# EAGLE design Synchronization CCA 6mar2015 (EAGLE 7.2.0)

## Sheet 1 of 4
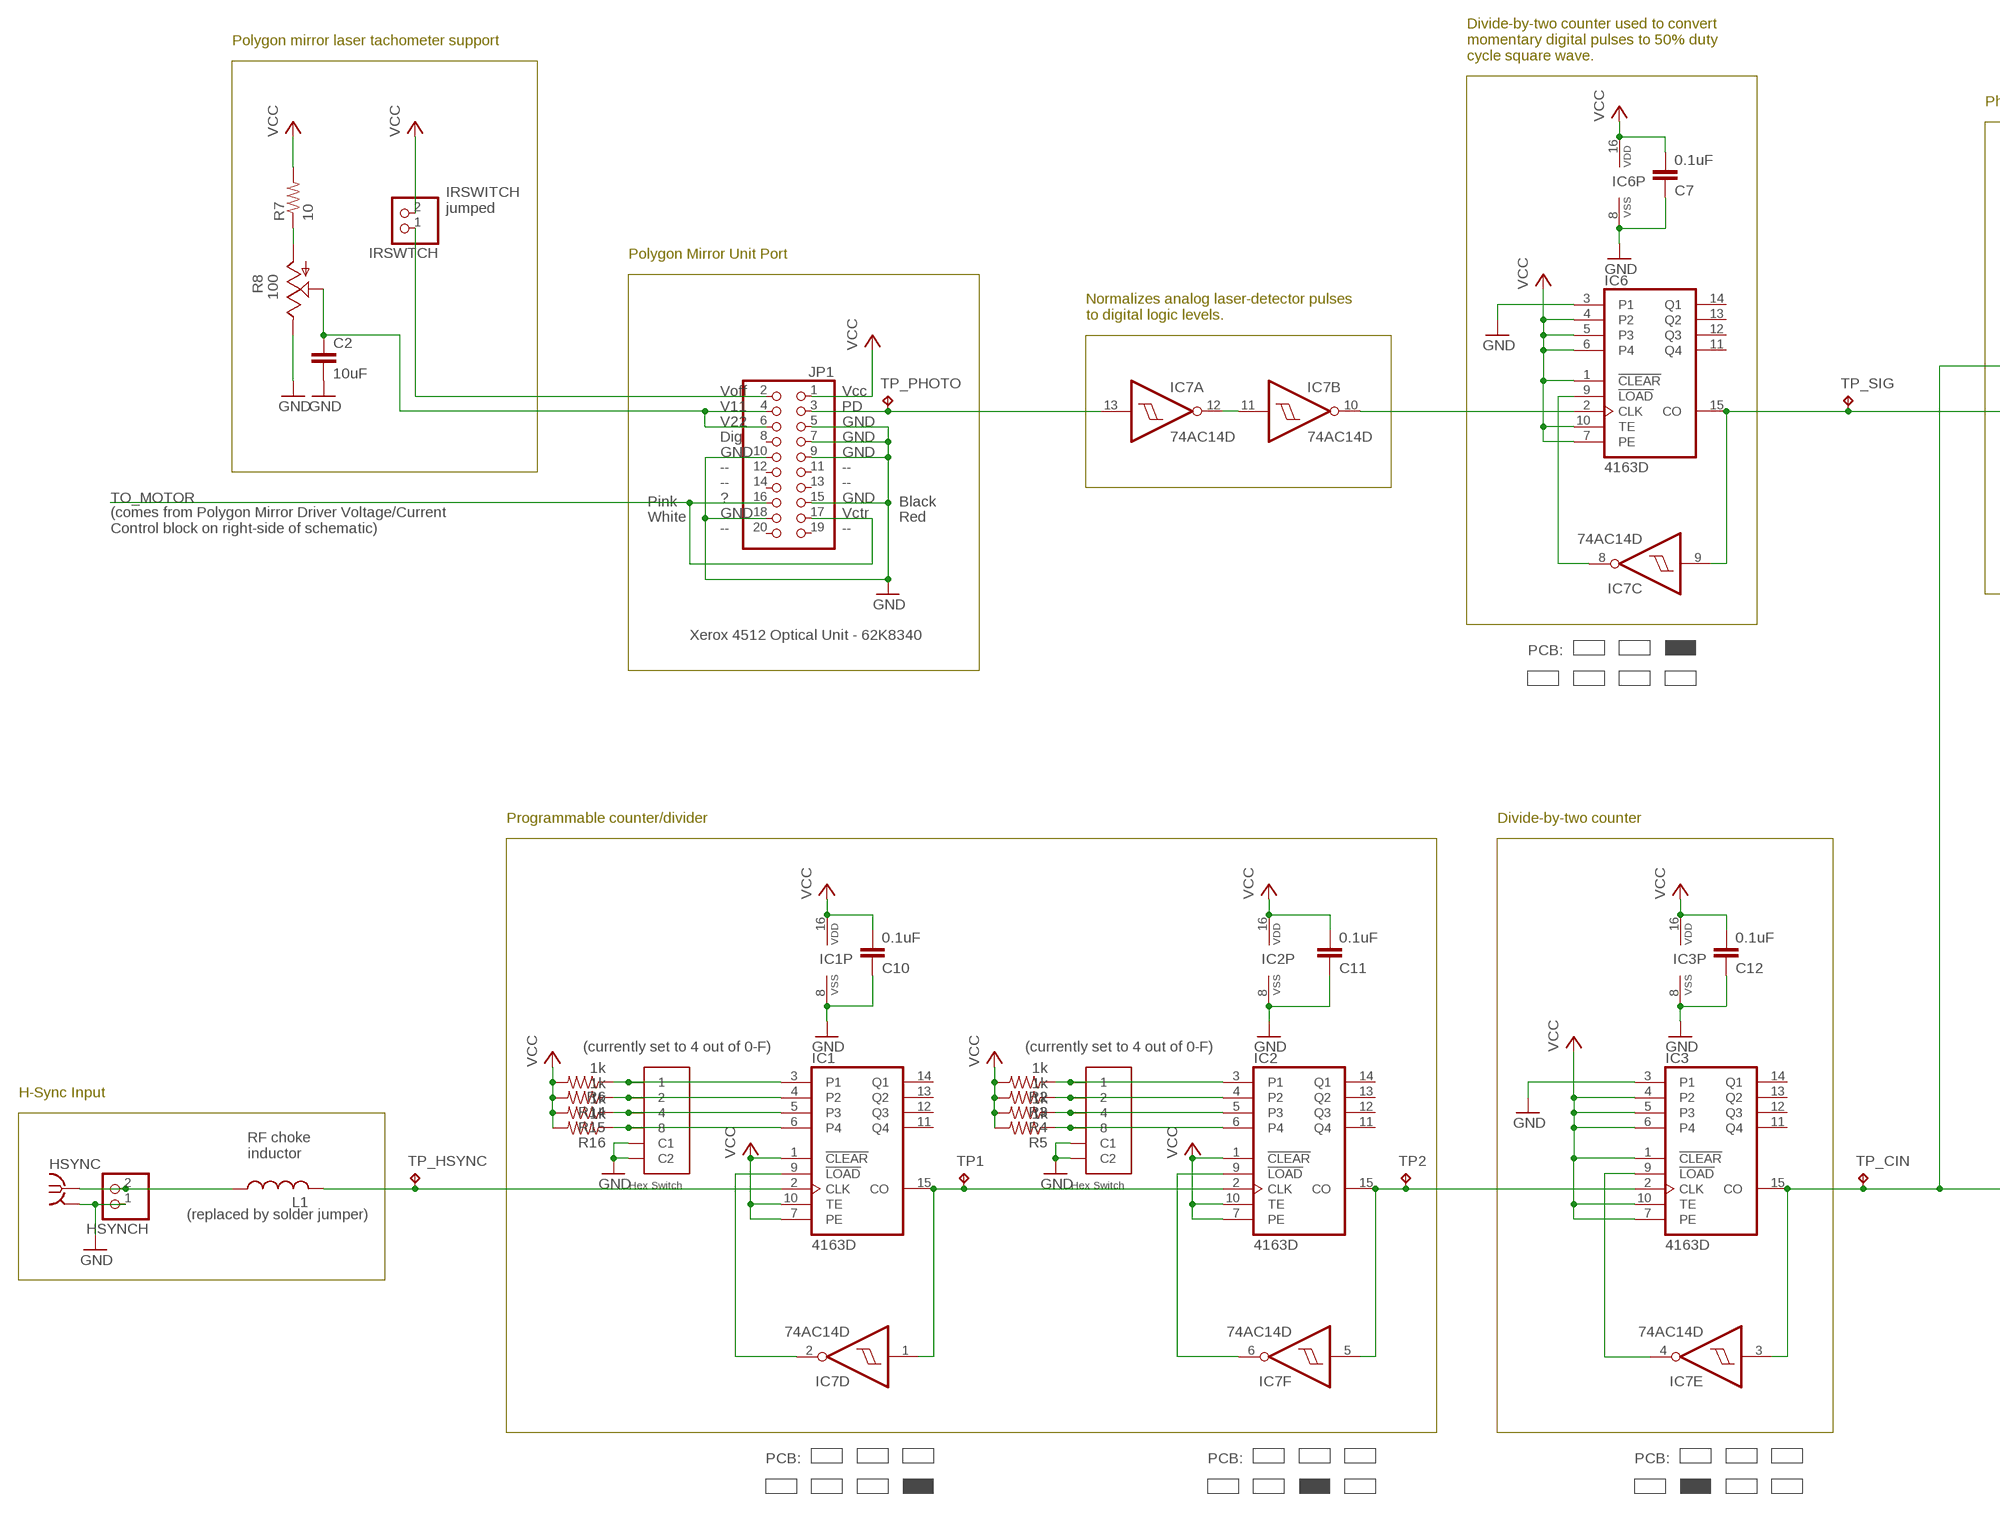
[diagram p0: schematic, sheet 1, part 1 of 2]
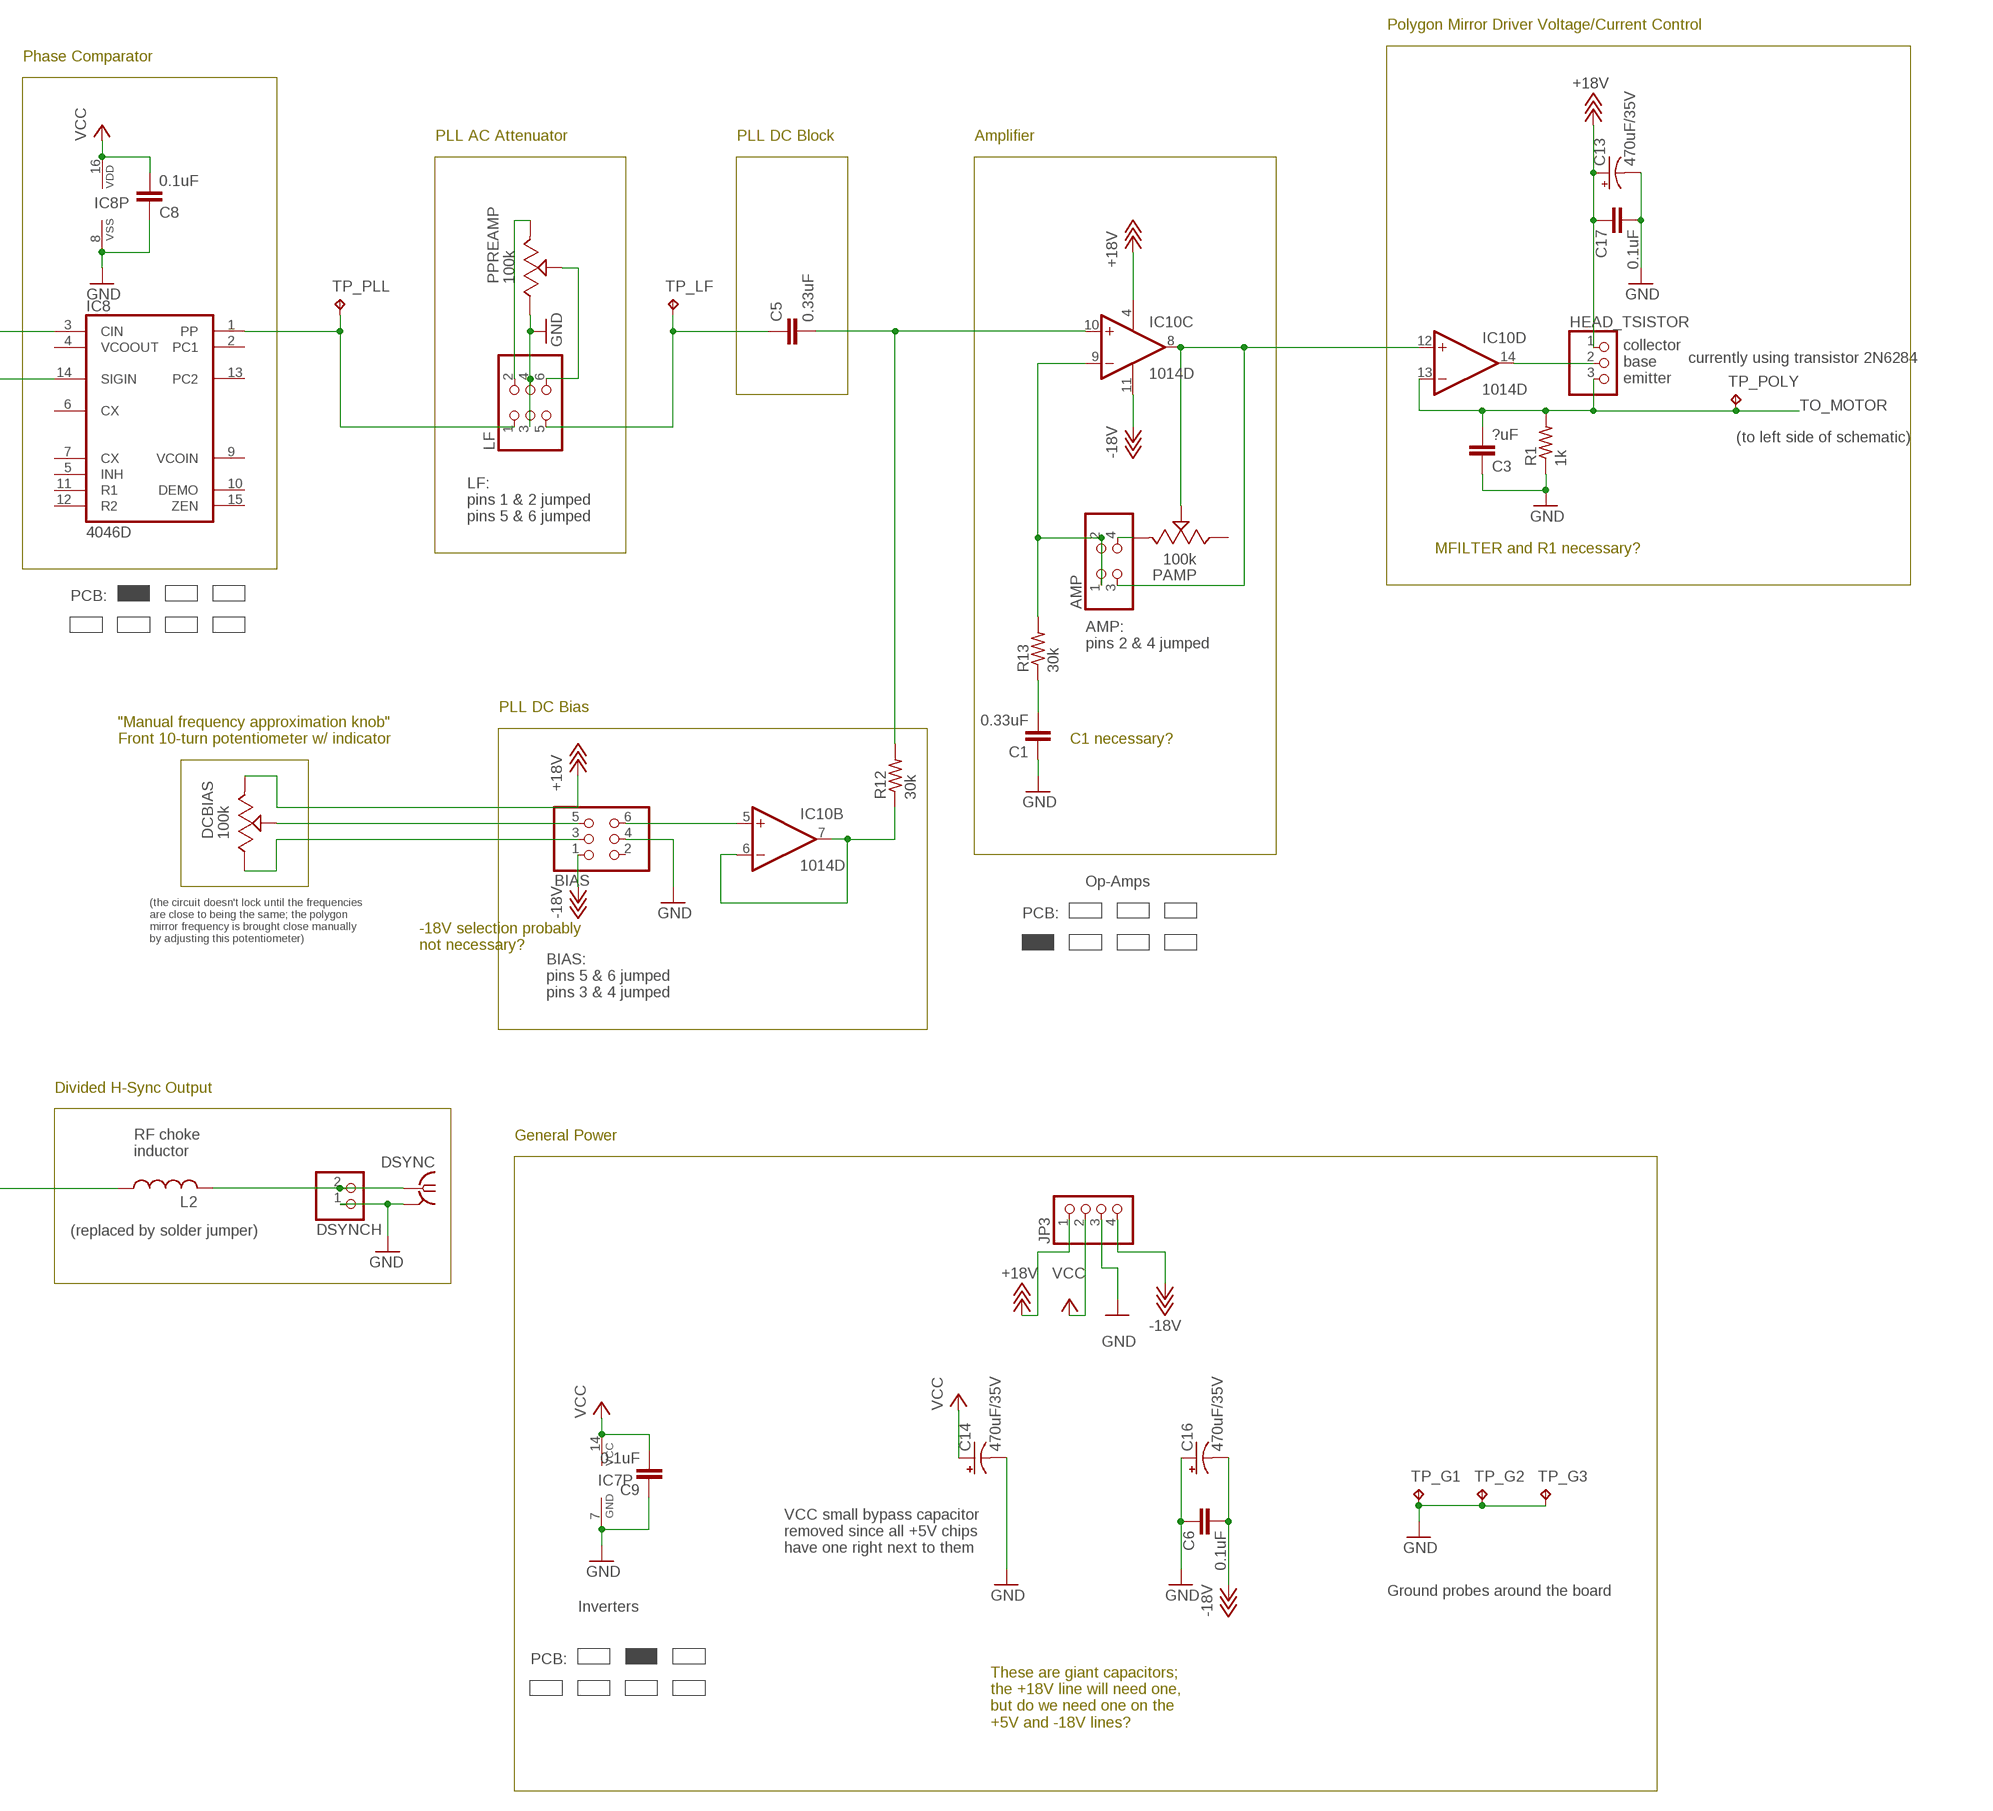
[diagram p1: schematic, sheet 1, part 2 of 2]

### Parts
AMP  PINHD-2X2  [2X02]
BIAS  PINHD-2X3  [2X03]
C1  0.33uF  C-EUC0805  [C0805]
C2  10uF  C-EUC0805  [C0805]
C3  ?uF  C-EUC0805  [C0805]
C5  0.33uF  C-EUC0805  [C0805]
C6  0.1uF  C-EUC0805  [C0805]
C7  0.1uF  C-EUC0805  [C0805]
C8  0.1uF  C-EUC0805  [C0805]
C9  0.1uF  C-EUC0805  [C0805]
C10  0.1uF  C-EUC0805  [C0805]
C11  0.1uF  C-EUC0805  [C0805]
C12  0.1uF  C-EUC0805  [C0805]
C13  470uF/35V  CPOL-USE5-10.5  [E5-10,5]
C14  470uF/35V  CPOL-USE5-10.5  [E5-10,5]
C16  470uF/35V  CPOL-USE5-10.5  [E5-10,5]
C17  0.1uF  C-EUC0805  [C0805]
DCBIAS  100k  POT3352  [POT3352]
DSYNC  SMA-142-0701-801/806  [J502-ND-142-0701-801/806]
DSYNCH  PINHD-1X2  [1X02]
HEAD_TSISTOR  PINHD-1X3  [1X03]
HEX1  HEXROTARY  [HEXROTARYP]
HEX2  HEXROTARY  [HEXROTARYP]
HSYNC  SMA-142-0701-801/806  [J502-ND-142-0701-801/806]
HSYNCH  PINHD-1X2  [1X02]
IC1  4163D  [SO16]
IC2  4163D  [SO16]
IC3  4163D  [SO16]
IC6  4163D  [SO16]
IC7  74AC14D  [SO14]
IC8  4046D  [SO16]
IC10  1014D  1014DDWD  [SO14]
IRSWTCH  PINHD-1X2  [1X02]
JP1  PINHD-2X10  [2X10]
JP3  PINHD-1X4  [1X04]
L1  L-USL2825P  [L2825P]
L2  L-USL2825P  [L2825P]
LF  PINHD-2X3  [2X03]
PAMP  100k  POT3352  [POT3352]
PPREAMP  100k  POT3352  [POT3352]
R1  1k  R-US_R0805  [R0805]
R2  1k  R-US_R0805  [R0805]
R3  1k  R-US_R0805  [R0805]
R4  1k  R-US_R0805  [R0805]
R5  1k  R-US_R0805  [R0805]
R6  1k  R-US_R0805  [R0805]
R7  10  R-US_R0805  [R0805]
R8  100  TRIM_US-S64W  [S64W]
R12  30k  R-US_R0805  [R0805]
R13  30k  R-US_R0805  [R0805]
R14  1k  R-US_R0805  [R0805]
R15  1k  R-US_R0805  [R0805]
R16  1k  R-US_R0805  [R0805]
TP1  TPTP11R  [TP11R]
TP2  TPTP11R  [TP11R]
TP_CIN  TPPAD1-17  [P1-17]
TP_G1  TPPAD1-17  [P1-17]
TP_G2  TPPAD1-17  [P1-17]
TP_G3  TPPAD1-17  [P1-17]
TP_HSYNC  TPPAD1-17  [P1-17]
TP_LF  TPPAD1-17  [P1-17]
TP_PHOTO  TPPAD1-17  [P1-17]
TP_PLL  TPPAD1-17  [P1-17]
TP_POLY  TPPAD1-17  [P1-17]
TP_SIG  TPPAD1-17  [P1-17]

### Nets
+18V: C13.+ C17.1 DCBIAS.P$3(E) HEAD_TSISTOR.1 IC10.4(P:V+) JP3.1
-18V: BIAS.1 C6.2 C16.- IC10.11(P:V-) JP3.4
GND: BIAS.4 C1.1 C2.2 C3.1 C6.1 C7.1 C8.1 C9.1 C10.1 C11.1 C12.1 C13.- C14.- C16.+ C17.2 DSYNC.G@1(GND) DSYNCH.1 HEX1.P$5(C1) HEX1.P$6(C2) HEX2.P$5(C1) HEX2.P$6(C2) HSYNC.G@1(GND) HSYNCH.1 IC1.8(VSS) IC2.8(VSS) IC3.3(P1) IC3.8(VSS) IC6.3(P1) IC6.8(VSS) IC7.7(P:GND) IC8.8(VSS) JP1.5 JP1.7 JP1.9 JP1.10 JP1.15 JP1.18 JP3.3 LF.3 LF.4 PPREAMP.P$1(A) R1.1 R8.E TP_G1.TP TP_G2.TP TP_G3.TP
HEX1: HEX1.P$2 IC1.4(P2) R14.1
HEX2: HEX2.P$2 IC2.4(P2) R3.1
N$1: IC1.9(!LOAD) IC7.2(D:O)
N$2: HEX1.P$1 IC1.3(P1) R6.1
N$3: IC1.15(CO) IC2.2(CLK) IC7.1(D:I) TP1.TP
N$4: IC2.9(!LOAD) IC7.6(F:O)
N$5: IC2.15(CO) IC3.2(CLK) IC7.5(F:I) TP2.TP
N$6: IC1.2(CLK) L1.2 TP_HSYNC.TP
N$7: IC3.15(CO) IC7.3(E:I) IC8.3(CIN) L2.1 TP_CIN.TP
N$8: IC3.9(!LOAD) IC7.4(E:O)
N$9: IRSWTCH.1 JP1.2
N$10: R7.1 R8.A
N$11: BIAS.5 DCBIAS.P$2(S)
N$12: BIAS.6 IC10.5(B:+IN)
N$13: HEX2.P$1 IC2.3(P1) R2.1
N$14: HEX1.P$3 IC1.5(P3) R15.1
N$15: HEX2.P$3 IC2.5(P3) R4.1
N$16: LF.2 PPREAMP.P$3(E)
N$18: IC10.6(B:-IN) IC10.7(B:OUT) R12.1
N$19: LF.6 PPREAMP.P$2(S)
N$20: HEX1.P$4 IC1.6(P4) R16.1
N$21: DSYNC.1 DSYNCH.2 L2.2
N$22: IC8.1(PP) LF.1 TP_PLL.TP
N$24: AMP.3 IC10.8(C:OUT) IC10.12(D:+IN) PAMP.P$2(S)
N$25: HEAD_TSISTOR.2 IC10.14(D:OUT)
N$26: HEX2.P$4 IC2.6(P4) R5.1
N$27: C5.1 LF.5 TP_LF.TP
N$28: IC7.13(A:I) JP1.3 TP_PHOTO.TP
N$29: AMP.1 AMP.2 IC10.9(C:-IN) R13.2
N$30: AMP.4 PAMP.P$3(E)
N$31: BIAS.3 DCBIAS.P$1(A)
N$32: HSYNC.1 HSYNCH.2 L1.1
N$33: IC7.11(B:I) IC7.12(A:O)
N$34: IC6.15(CO) IC7.9(C:I) IC8.14(SIGIN) TP_SIG.TP
N$35: IC6.9(!LOAD) IC7.8(C:O)
N$37: C5.2 IC10.10(C:+IN) R12.2
N$38: C1.2 R13.1
N$40: IC6.2(CLK) IC7.10(B:O)
TO_LASER: C2.1 JP1.4 JP1.6 R8.S
TO_MOTOR: C3.2 HEAD_TSISTOR.3 IC10.13(D:-IN) JP1.16 JP1.17 R1.2 TP_POLY.TP
VCC: C7.2 C8.2 C9.2 C10.2 C11.2 C12.2 C14.+ IC1.1(!CLEAR) IC1.7(PE) IC1.10(TE) IC1.16(VDD) IC2.1(!CLEAR) IC2.7(PE) IC2.10(TE) IC2.16(VDD) IC3.1(!CLEAR) IC3.4(P2) IC3.5(P3) IC3.6(P4) IC3.7(PE) IC3.10(TE) IC3.16(VDD) IC6.1(!CLEAR) IC6.4(P2) IC6.5(P3) IC6.6(P4) IC6.7(PE) IC6.10(TE) IC6.16(VDD) IC7.14(P:VCC) IC8.16(VDD) IRSWTCH.2 JP1.1 JP3.2 R2.2 R3.2 R4.2 R5.2 R6.2 R7.2 R14.2 R15.2 R16.2
Unconnected: BIAS.2 IC1.11(Q4) IC1.12(Q3) IC1.13(Q2) IC1.14(Q1) IC2.11(Q4) IC2.12(Q3) IC2.13(Q2) IC2.14(Q1) IC3.11(Q4) IC3.12(Q3) IC3.13(Q2) IC3.14(Q1) IC6.11(Q4) IC6.12(Q3) IC6.13(Q2) IC6.14(Q1) IC8.2(PC1) IC8.4(VCOOUT) IC8.5(INH) IC8.6(CX) IC8.7(CX) IC8.9(VCOIN) IC8.10(DEMO) IC8.11(R1) IC8.12(R2) IC8.13(PC2) IC8.15(ZEN) IC10.1(A:OUT) IC10.2(A:-IN) IC10.3(A:+IN) JP1.8 JP1.11 JP1.12 JP1.13 JP1.14 JP1.19 JP1.20 PAMP.P$1(A)

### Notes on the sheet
- Polygon mirror laser tachometer support
- Divide-by-two counter used to convert
  momentary digital pulses to 50% duty
  cycle square wave.
- Polygon Mirror Driver Voltage/Current Control
- Phase Comparator
- PLL AC Attenuator | PLL DC Block | Amplifier
- IRSWITCH
  jumped
- Polygon Mirror Unit Port
- Normalizes analog laser-detector pulses
  to digital logic levels.
- Voff | Vcc | currently using transistor 2N6284
- V11 | PD
- collector
  base
  emitter
- V22 | GND
- Dig | GND
- GND | GND
- -- | -- | (to left side of schematic)
- -- | --
- Pink | ? | GND | Black
- White | GND | Vctr | Red
- (comes from Polygon Mirror Driver Voltage/Current
  Control block on right-side of schematic)
- -- | --
- LF:
  pins 1 & 2 jumped
  pins 5 & 6 jumped
- MFILTER and R1 necessary?
- PCB:
- Xerox 4512 Optical Unit - 62K8340
- PCB:
- AMP:
  pins 2 & 4 jumped
- PLL DC Bias
- "Manual frequency approximation knob"
  Front 10-turn potentiometer w/ indicator
- C1 necessary?
- Programmable counter/divider | Divide-by-two counter
- Op-Amps
- PCB:
- (the circuit doesn't lock until the frequencies
  are close to being the same; the polygon
  mirror frequency is brought close manually
  by adjusting this potentiometer)
- -18V selection probably
  not necessary?
- BIAS:
  pins 5 & 6 jumped
  pins 3 & 4 jumped
- (currently set to 4 out of 0-F) | (currently set to 4 out of 0-F)
- H-Sync Input | Divided H-Sync Output
- General Power
- RF choke
  inductor
- RF choke
  inductor
- (replaced by solder jumper)
- (replaced by solder jumper)
- PCB: | PCB: | PCB:
- VCC small bypass capacitor
  removed since all +5V chips
  have one right next to them
- Ground probes around the board
- Inverters
- PCB:
- These are giant capacitors;
  the +18V line will need one,
  but do we need one on the
  +5V and -18V lines?

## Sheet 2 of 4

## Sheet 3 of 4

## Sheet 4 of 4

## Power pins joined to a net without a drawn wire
GND: DSYNC.G@2(GND) DSYNC.G@3(GND) DSYNC.G@4(GND) HSYNC.G@2(GND) HSYNC.G@3(GND) HSYNC.G@4(GND)

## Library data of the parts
AMP = pinhead:PINHD-2X2: PIN HEADER
BIAS LF = pinhead:PINHD-2X3: PIN HEADER
C1-C3 C5-C12 C17 = rcl:C-EU: CAPACITOR, European symbol
C13 C14 C16 = rcl:CPOL-US: POLARIZED CAPACITOR, American symbol
DCBIAS PAMP PPREAMP = Daniel:POT3352: 3352 potentiometer
DSYNC HSYNC = con-coax:SMA-: SMA 50 Ohm End Launch Jack Receptacle - Round Contact Johnson Components Source: www.johnsoncomponents.com .. J502-ND.pdf; MF: JOHNSON COMPONENTS; MPN: 142-0701-801; OC_FARNELL: 1608592; OC_NEWARK: 90F2624
DSYNCH HSYNCH IRSWTCH = pinhead:PINHD-1X2: PIN HEADER
HEAD_TSISTOR = pinhead:PINHD-1X3: PIN HEADER
HEX1 HEX2 = Danhex:HEXROTARY
IC1-IC3 IC6 = 40xx:4163: Synchronous presettable 4-bit binary COUNTER
IC7 = 74xx-eu:74*14: Hex schmitt trigger INVERTER
IC8 = 40xx:4046: Micropower PLL
IC10 = Daniel:1014DDW: Quad Op Amp general purpose 1014 uses a wide range of supply voltages up to 30V
JP1 = pinhead:PINHD-2X10: PIN HEADER
JP3 = pinhead:PINHD-1X4: PIN HEADER
L1 L2 = rcl:L-US: INDUCTOR, American symbol
R1-R7 R12-R16 = rcl:R-US_: RESISTOR, American symbol
R8 = pot:TRIM_US-: POTENTIOMETER
TP1 TP2 TP_CIN TP_G1-TP_G3 TP_HSYNC TP_LF TP_PHOTO TP_PLL TP_POLY TP_SIG = testpad:TP: Test pad

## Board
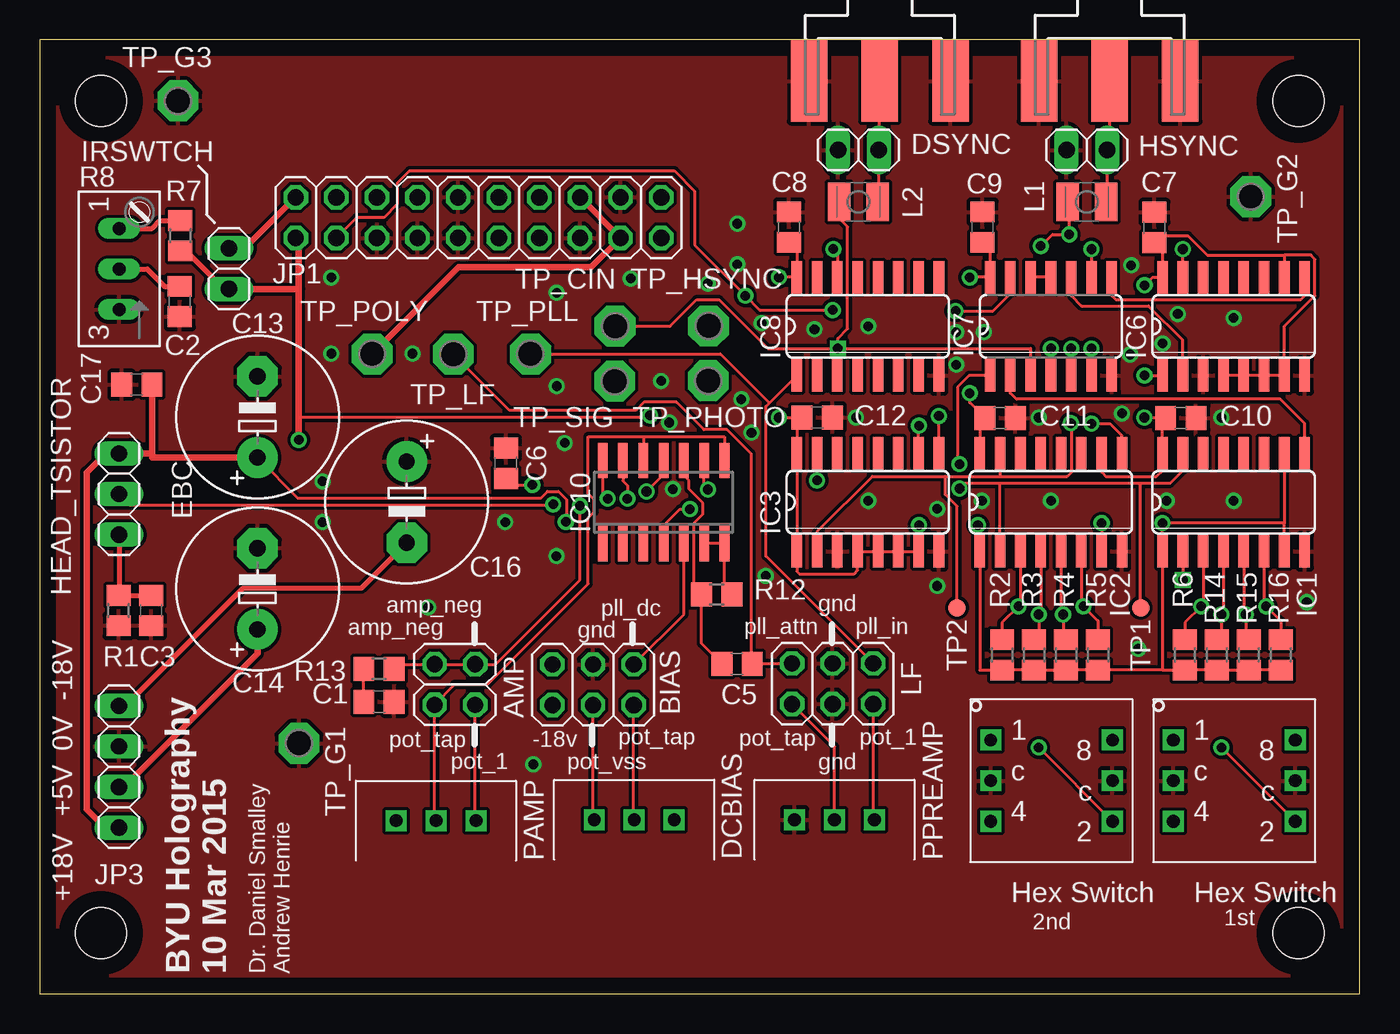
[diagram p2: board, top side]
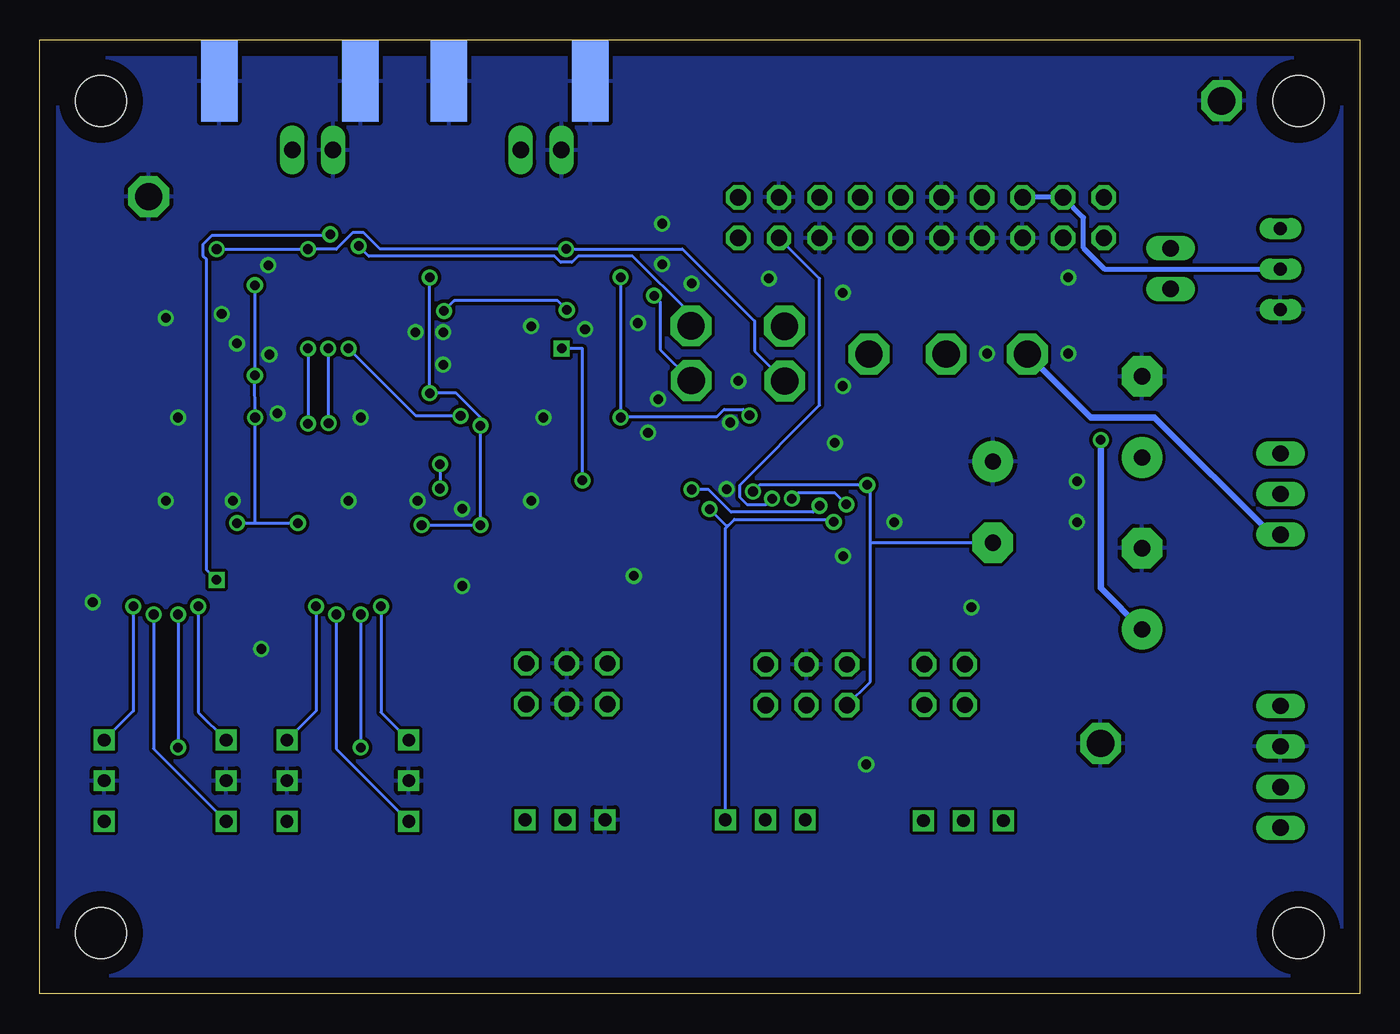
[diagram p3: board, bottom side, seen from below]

Size 82.55 x 59.69 mm. Coordinates in mm from the lower left corner, seen from the top.
Outline: 0,0 82.55,0 82.55,59.69 0,59.69 0,0
Copper layers (1*16): Top 0.035mm / dielectric 1.5mm / Bottom 0.035mm
Design rules "default *": minimum track width 10mil, minimum drill 24mil, track to track 8mil, track to pad 8mil, pad to pad 8mil, via to via 8mil, smd to smd 8mil, copper to edge 40mil, drill to drill 8mil, minimum pad ring 10mil, minimum via ring 8mil, stop-mask expansion 4mil, vias tented up to drill 25mil, thermal gap 10mil
Holes 3.2 mm at 3.81,55.88 78.74,55.88 78.74,3.81 3.81,3.81

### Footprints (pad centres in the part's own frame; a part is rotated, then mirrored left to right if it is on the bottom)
2X02 = drill 1.016 octagon: 1 -1.27,-1.27; 2 -1.27,1.27; 3 1.27,-1.27; 4 1.27,1.27
2X03 = drill 1.016 octagon: 1 -2.54,-1.27; 2 -2.54,1.27; 3 0,-1.27; 4 0,1.27; 5 2.54,-1.27; 6 2.54,1.27
C0805 = smd 1.3 x 1.5: 1 -0.95,0; 2 0.95,0
E5-10,5 = drill 1.016 pad 2.54: + -2.54,0 | drill 1.016 pad 2.54 octagon: - 2.54,0
POT3352 = drill 0.8 square: P$1 -2.5,0; P$2 0,0; P$3 2.5,0
J502-ND-142-0701-801/806 = smd 5.08 x 2.286: 1 2.565,0; G@1 2.565,4.42; G@2 2.565,-4.42 | smd 5.08 x 2.286 bottom: G@3 2.565,4.42; G@4 2.565,-4.42
1X02 = drill 1.016 long: 1 -1.27,0; 2 1.27,0
1X03 = drill 1.016 long: 1 -2.54,0; 2 0,0; 3 2.54,0
HEXROTARYP = drill 0.8 square: P$1 -11.43,7.62; P$2 -3.81,2.54; P$3 -11.43,2.54; P$4 -3.81,7.62; P$5 -11.43,5.08; P$6 -3.81,5.08
SO16 = smd 0.66 x 2.032: 1 -4.445,-3.073; 2 -3.175,-3.073; 3 -1.905,-3.073; 4 -0.635,-3.073; 5 0.635,-3.073; 6 1.905,-3.073; 7 3.175,-3.073; 8 4.445,-3.073; 9 4.445,3.073; 10 3.175,3.073; 11 1.905,3.073; 12 0.635,3.073; 13 -0.635,3.073; 14 -1.905,3.073; 15 -3.175,3.073; 16 -4.445,3.073
SO14 = smd 0.66 x 2.032: 1 -3.81,-3.073; 2 -2.54,-3.073; 3 -1.27,-3.073; 4 0,-3.073; 5 1.27,-3.073; 6 2.54,-3.073; 7 3.81,-3.073; 8 3.81,3.073; 9 2.54,3.073; 10 1.27,3.073; 11 0,3.073; 12 -1.27,3.073; 13 -2.54,3.073; 14 -3.81,3.073
SO14' = smd 0.6 x 2.2: 1 -3.81,-2.6; 2 -2.54,-2.6; 3 -1.27,-2.6; 4 0,-2.6; 5 1.27,-2.6; 6 2.54,-2.6; 7 3.81,-2.6; 8 3.81,2.6; 9 2.54,2.6; 10 1.27,2.6; 11 0,2.6; 12 -1.27,2.6; 13 -2.54,2.6; 14 -3.81,2.6
2X10 = drill 1.016 octagon: 1 -11.43,-1.27; 2 -11.43,1.27; 3 -8.89,-1.27; 4 -8.89,1.27; 5 -6.35,-1.27; 6 -6.35,1.27; 7 -3.81,-1.27; 8 -3.81,1.27; 9 -1.27,-1.27; 10 -1.27,1.27; 11 1.27,-1.27; 12 1.27,1.27; 13 3.81,-1.27; 14 3.81,1.27; 15 6.35,-1.27; 16 6.35,1.27; 17 8.89,-1.27; 18 8.89,1.27; 19 11.43,-1.27; 20 11.43,1.27
1X04 = drill 1.016 long: 1 -3.81,0; 2 -1.27,0; 3 1.27,0; 4 3.81,0
L2825P = smd 1.4 x 2.4: 1 -1.2,0; 2 1.2,0
R0805 = smd 1.3 x 1.5: 1 -0.95,0; 2 0.95,0
S64W = drill 0.813 long: A 2.54,1.27; E -2.54,1.27; S 0,1.27
TP11R = smd 1.1 x 1.1: TP 0,0
P1-17 = drill 1.702 pad 2.54 octagon: TP 0,0

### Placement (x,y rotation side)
AMP  25.95,19.36 270 top
BIAS  34.6,19.35 0 top
C1  21.21,18.29 180 top
C2  8.75,43.32 270 top
C3  6.95,23.99 90 top
C5  43.61,20.65 180 top
C6  29.15,33.21 270 top
C7  69.72,47.96 270 top
C8  46.86,47.98 270 top
C9  58.96,47.98 270 top
C10  71.37,36.04 180 top
C11  60.07,36.04 180 top
C12  48.63,36.07 180 top
C13  13.61,36.11 90 top
C14  13.61,25.35 90 top
C16  22.94,30.77 270 top
C17  6.06,38.12 180 top
DCBIAS  37.18,10.9 0 top
DSYNC  52.54,59.69 270 top
DSYNCH  51.2,52.8 0 top
HEAD_TSISTOR  4.95,31.28 270 top
HEX1  82.34,8.27 0 top
HEX2  70.91,8.27 0 top
HSYNC  66.91,59.69 270 top
HSYNCH  65.49,52.8 0 top
IC1  74.67,30.77 0 top
IC2  63.24,30.77 0 top
IC3  51.79,30.77 0 top
IC6  74.67,41.77 0 top
IC7  63.24,41.77 0 top
IC8  51.79,41.77 0 top
IC10  1014D  [SO14']  39.01,30.77 0 top
IRSWTCH  11.83,45.38 270 top
JP1  27.43,48.57 0 top
JP3  4.95,14.22 90 top
L1  65.49,49.56 180 top
L2  51.2,49.56 0 top
LF  49.59,19.41 180 top
PAMP  24.78,10.84 0 top
PPREAMP  49.7,10.9 0 top
R1  4.92,23.99 90 top
R2  60.19,21.21 270 top
R3  62.19,21.21 270 top
R4  64.19,21.21 270 top
R5  66.19,21.21 270 top
R6  71.62,21.21 270 top
R7  8.78,47.44 270 top
R8  6.22,45.36 90 top
R12  42.34,25 180 top
R13  21.21,20.34 0 top
R14  73.62,21.21 270 top
R15  75.62,21.21 270 top
R16  77.62,21.21 270 top
TP1  68.86,24.15 270 top
TP2  57.37,24.15 270 top
TP_CIN  35.98,41.78 270 top
TP_G1  16.2,15.68 0 top
TP_G2  75.75,49.89 90 top
TP_G3  8.64,55.88 0 top
TP_HSYNC  41.83,41.8 270 top
TP_LF  25.86,40.03 270 top
TP_PHOTO  41.8,38.37 270 top
TP_PLL  30.68,40.04 270 top
TP_POLY  20.78,40.04 270 top
TP_SIG  35.96,38.34 270 top

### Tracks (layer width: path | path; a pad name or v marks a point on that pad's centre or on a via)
+18V  (via drill 0.6)
  Top 0.203: IC10.4 39.01,29.3 40.04,30.33 v40.65,30.33 | C13.+ 16.16,31.01 31.32,31.01 31.75,31.45 32.44,31.45 32.96,30.92 32.96,29.6 v32.89,29.54
  Top 0.406: 7.01,33.82 HEAD_TSISTOR.1 4.1,33.82 2.92,32.64 2.92,11.56 4.07,10.41 JP3.1 | 7.01,33.82 C17.1 | C13.+ 7.01,33.56 7.01,33.82
  Bottom 0.203: DCBIAS.P$3 39.68,29.13 39.48,29.32 | 39.48,29.32 39.12,29.69 33.05,29.69 v32.89,29.54 | v40.65,30.33 39.64,29.32 39.48,29.32
-18V  (via drill 0.6)
  Top 0.203: v37.95,31.44 39.01,32.5 IC10.11 | C6.2 29.55,31.85 v30.8,31.85
  Top 0.305: JP3.4 5.33,18.03 12.7,25.4 20.11,25.4 C16.-
  Bottom 0.203: BIAS.1 30.61,19.53 30.61,28.23 | 30.61,28.23 30.61,31.66 v30.8,31.85 37.53,31.85 v37.95,31.44 | C16.- 30.61,28.23
GND  (via drill 0.6)
  other vias: 73.91,36.07 62.48,36.07 51.05,36.07 74.68,30.86 74.68,42.29 59.05,41.4 63.25,30.86 51.82,30.86 51.82,41.78 68.2,40.01 57.33,39.37 67.69,36.32 56.13,30.35 58.93,30.86 70.48,30.86 68.26,45.59 68.71,21.59 56.13,25.53 79.25,24.51 23.3,40.07 32.31,27.39 24.28,24.19 18.22,40.07 32.32,43.88 38.86,38.35 45.15,41.97 36.96,44.77 43.62,45.66 44.51,35.12 71.18,42.55 70.23,40.7 57.33,41.4 48.45,41.59 43.88,37.21 41.78,44.45 39.37,35.75 45.4,26.16 39.6,31.58 30.86,14.36 18.22,44.83 32.32,38.04 32.83,34.48 43.62,48.2 29.11,29.53 17.68,29.53 17.68,32.07
  pour Top: 0,59.69 82.55,59.69 82.55,0 0,0
  pour Bottom: 0,59.69 0,0 82.55,0 82.55,59.69
HEX1  (via drill 0.6)
  Top 0.203: IC1.4 74.03,23.87 v73.91,23.75 73.91,22.45 R14.1 | v73.91,15.42 HEX1.P$2
  Bottom 0.203: v73.91,23.75 v73.91,15.42
HEX2  (via drill 0.6)
  Top 0.203: IC2.4 62.6,23.87 v62.48,23.75 62.48,22.45 R3.1 | v62.48,15.42 HEX2.P$2
  Bottom 0.203: v62.48,23.75 v62.48,15.42
N$1
  Top 0.203: IC1.9 79.11,35.69 77.6,37.21 61.09,37.21 60.71,37.59 IC7.2
N$2  (via drill 0.6)
  Top 0.203: IC1.3 72.77,24.38 v72.64,24.26 71.62,23.23 R6.1
  Bottom 0.203: v72.64,24.26 72.64,17.62 HEX1.P$1
N$3  (via drill 0.6)
  Top 0.203: IC1.15 71.5,32.76 70.67,31.94 68.83,31.94 | IC7.1 58.12,38.69 57.4,37.97 57.4,33.27 v57.53,33.15 | 68.83,31.94 60.06,31.94 | 60.06,31.94 57.85,31.94 v57.53,31.62 | IC2.2 60.06,31.94 | TP1.TP 68.83,24.31 68.83,31.94
  Bottom 0.203: v57.53,33.15 v57.53,31.62
N$4  (via drill 0.6)
  Top 0.203: IC7.6 v65.78,40.39 | IC2.9 67.69,34.93 66.93,35.69 v65.78,35.69
  Bottom 0.203: v65.78,40.39 v65.78,35.69
N$5  (via drill 0.6)
  Top 0.203: v64.52,40.39 IC7.5 | v64.49,35.71 64.52,35.69 64.52,32.64 64.26,32.38 60.06,32.38 | IC3.2 48.62,28.93 52.07,32.38 56.64,32.38 | 56.64,32.38 60.06,32.38 | IC2.15 60.06,32.38 | TP2.TP 57.37,30.52 56.64,31.24 56.64,32.38
  Bottom 0.203: v64.49,35.71 64.49,40.39 v64.52,40.39
N$6  (via drill 0.6)
  Top 0.203: IC1.2 v71.5,25.91 | L1.2 64.39,49.46 v64.39,47.52 63.34,47.52 v62.61,46.8
  Bottom 0.203: v71.5,25.91 72.14,26.54 72.14,45.97 72.33,46.16 72.33,46.93 71.78,47.47 64.44,47.47 v64.39,47.52 | TP_HSYNC.TP 41.83,42.53 45.47,46.16 48.9,46.16 49.28,45.78 49.97,45.78 50.35,46.16 61.98,46.16 v62.61,46.8
N$7  (via drill 0.6)
  Top 0.203: IC3.15 v48.62,32.13 | 49.91,38.73 IC8.3 49.89,40.36 v49.91,40.39 | v49.91,40.39 61.97,40.39 | 61.97,40.39 61.98,40.39 | IC7.3 61.97,40.39 | v49.91,40.39 49.91,41.02 50.52,41.63 50.52,48 50,48.52 L2.1 | TP_CIN.TP 39.43,41.78 41.08,43.43 42.48,43.43 45.53,40.39 v49.91,40.39
  Bottom 0.203: v48.62,32.13 48.62,40.39 v49.91,40.39
N$8  (via drill 0.6)
  Top 0.203: IC7.4 v63.24,40.38 v63.25,40.39 | IC3.9 v56.24,36.17
  Bottom 0.203: v56.24,36.17 59.03,36.17 v63.25,40.39
N$9
  Top 0.406: IRSWTCH.1 12.81,46.65 JP1.2
N$10
  Top 0.305: R8.A 7.01,47.9 7.5,48.39 R7.1
N$11
  Top 0.203: DCBIAS.P$2 37.14,10.94 BIAS.5
N$12
  Top 0.203: BIAS.6 40.28,23.76 IC10.5
N$13  (via drill 0.6)
  Top 0.203: IC2.3 61.34,24.38 v61.21,24.26 60.19,23.23 R2.1
  Bottom 0.203: v61.21,24.26 61.21,17.62 HEX2.P$1
N$14  (via drill 0.6)
  Top 0.203: IC1.5 75.31,23.88 v75.44,23.75 75.44,22.34 R15.1
  Bottom 0.203: v75.44,23.75 75.44,15.34 HEX1.P$3
N$15  (via drill 0.6)
  Top 0.203: IC2.5 63.88,23.88 v64.01,23.75 64.01,22.34 R4.1
  Bottom 0.203: v64.01,23.75 64.01,15.34 HEX2.P$3
N$16
  Top 0.203: PPREAMP.P$3 52.13,10.98 LF.2
N$18
  Top 0.203: R12.1 42.82,25.47 IC10.7 IC10.6
N$19
  Top 0.203: PPREAMP.P$2 49.7,15.48 LF.6
N$20  (via drill 0.6)
  Top 0.203: IC1.6 76.58,24.39 v76.71,24.26 77.62,23.34 R16.1
  Bottom 0.203: v76.71,24.26 76.71,17.7 HEX1.P$4
N$21
  Top 0.203: DSYNC.1 52.47,57.01 DSYNCH.2 52.47,49.62 L2.2
N$22
  Top 0.203: IC8.1 45.63,36.98 | 45.63,36.98 45.4,36.76 45.4,27.4 LF.1 | TP_PLL.TP 42.57,40.04 45.63,36.98
N$24
  Top 0.203: PAMP.P$2 24.68,10.94 AMP.3 25.95,19.36 27.99,19.36 34.29,25.65 34.29,29.79 34.67,30.17 34.67,30.93 34.29,31.31 34.29,34.87 37.74,34.87 | 37.74,34.87 IC10.12 | 37.74,34.87 42.82,34.87 IC10.8
N$25  (via drill 0.6)
  Top 0.203: IC10.14 35.2,31.3 v35.51,30.99 | HEAD_TSISTOR.2 5.62,30.61 32.08,30.61 v32.11,30.63
  Bottom 0.203: v35.51,30.99 35.1,31.37 32.84,31.37 v32.11,30.63
N$26  (via drill 0.6)
  Top 0.203: IC2.6 65.14,24.39 v65.28,24.26 66.19,23.34 R5.1
  Bottom 0.203: v65.28,24.26 65.28,17.7 HEX2.P$4
N$27
  Top 0.203: LF.5 44.58,20.68 C5.1 44.49,20.72 44.49,33.8 42.99,35.31 41.53,35.31 39.81,37.02 37.78,37.02 37.27,36.51 29.38,36.51 TP_LF.TP
N$28  (via drill 0.6)
  Top 0.203: v49.59,42.8 45.02,42.8 v44.13,43.69 40.96,46.86 40.96,50.23 39.69,51.5 23.12,51.5 22.35,50.73 22.35,49.4 21.53,48.58 19.82,48.58 JP1.3 | IC7.13 60.71,43.81 59.63,42.74 v57.28,42.74
  Bottom 0.203: TP_PHOTO.TP 43.75,40.32 43.75,43.31 v44.13,43.69 | v49.59,42.8 50.16,43.37 56.64,43.37 v57.28,42.74
N$29  (via drill 0.6)
  Top 0.203: R13.2 22.45,20.63 AMP.1 AMP.2 28.51,20.63 33.78,25.91 v33.78,30.55 | v41.78,31.57 41.55,31.8 IC10.9
  Bottom 0.203: v33.78,30.55 34.19,30.14 39.32,30.14 40.74,31.57 v41.78,31.57
N$30
  Top 0.203: PAMP.P$3 27.23,10.89 AMP.4
N$31
  Top 0.203: DCBIAS.P$1 34.6,10.98 BIAS.3
N$32
  Top 0.203: HSYNC.1 66.89,52.93 HSYNCH.2 66.76,49.62 L1.1
N$33
  Top 0.203: IC7.11 IC7.12
N$34  (via drill 0.6)
  Top 0.203: IC6.15 v71.5,46.6 | v65.78,46.6 IC7.9 | v49.63,46.61 49.89,46.35 IC8.14
  Bottom 0.203: v71.5,46.6 v65.78,46.6 64.01,46.6 62.99,47.62 62.29,47.62 61.28,46.61 v49.63,46.61 | v49.63,46.61 v49.63,46.6 | v49.63,46.61 42.35,46.61 37.85,42.1 37.85,40.23 TP_SIG.TP
N$35
  Top 0.203: IC7.8 67.05,43.69 67.31,43.43 78.87,43.43 79.12,43.69 IC6.9
N$37
  Top 0.203: IC10.10 40.28,32.43 40.59,32.12 40.59,31.6 41.48,30.71 41.48,30.02 40.92,29.46 40.92,25.47 R12.2 41.39,21.92 C5.2
N$38
  Top 0.203: C1.2 R13.1
N$40
  Top 0.203: IC7.10 64.51,43.69 65.15,43.05 69.34,43.05 71.5,40.9 IC6.2
TO_LASER
  Top 0.305: R8.S 6.71,45.36 7.8,44.27 C2.1
  Bottom 0.305: JP1.6 JP1.4 17.27,48.57 17.27,46.67 15.96,45.36 R8.S
TO_MOTOR  (via drill 0.6)
  Top 0.203: IC10.13 36.47,32.11 36.75,31.83 v36.75,30.99
  Top 0.305: HEAD_TSISTOR.3 4.95,24.97 R1.2 C3.2
  Top 0.406: TP_POLY.TP 26.2,45.47 34.48,45.47 JP1.17 JP1.16
  Bottom 0.203: v36.75,30.99 37.13,30.61 38.3,30.61 38.77,31.08 38.77,31.84 33.78,36.83 33.78,44.76 JP1.17
  Bottom 0.406: HEAD_TSISTOR.3 5.5,28.74 12.83,36.07 16.8,36.07 TP_POLY.TP
VCC  (via drill 0.6)
  Top 0.203: R16.2 R15.2 R14.2 R6.2 70.22,20.26 | IC6.4 IC6.5 IC6.6 IC6.7 77.84,41.78 79.76,43.69 79.76,45.97 79.5,46.23 77.85,46.23 | C7.2 70.22,47.01 | 70.22,47.01 IC6.16 69.61,44.85 v69.1,44.34 | IC2.10 66.42,32.65 66.67,32.38 69.85,32.38 70.23,32.77 IC1.16 70.22,36.04 C10.2 70.42,36.07 v69.09,36.07 | v69.1,38.7 IC6.1 | v66.42,29.46 IC2.7 | 70.22,20.26 IC1.1 v70.22,29.46 77.84,29.46 | 70.22,20.26 R5.2 R4.2 R3.2 R2.2 58.8,20.26 IC2.1 58.8,29.22 v58.67,29.34 | IC2.16 58.8,35.72 C11.2 58.17,37 v58.17,37.59 | v46.23,44.85 IC8.16 47.35,46.54 C8.2 | v46.23,36.07 C12.2 47.35,35.74 IC3.16 IC3.1 47.35,26.44 47.5,26.29 50.93,26.29 51.16,26.52 IC3.4 IC3.5 IC3.6 IC3.7 54.97,29.31 v54.99,29.34 | 58.18,44.85 v58.17,44.83 arc-90 58.18,44.85 | IC3.10 54.97,35.53 v54.99,35.56 | IC1.7 77.84,29.46 | IC1.10 77.84,29.46 | 77.85,46.23 IC6.10 | 77.85,46.23 73.03,46.23 71.82,47.43 70.22,47.43 70.22,47.01 | 58.18,44.85 IC7.14 59.43,46.56 C9.2 | v38.16,36.2 38.04,36.07 16.19,36.07 16.19,35.94
  Top 0.305: 11.51,44.11 9.14,46.49
  Top 0.406: JP3.2 5.26,12.95 13.61,21.29 C14.+ | v16.19,34.67 16.19,35.94 16.19,44.11 | 16.19,44.11 16.19,47.11 JP1.1 | 16.19,44.11 IRSWTCH.2 11.51,44.11 | 9.14,46.49 R7.2
  Bottom 0.203: v69.1,44.34 v69.1,38.7 v69.09,36.07 69.09,29.46 | v70.22,29.46 69.09,29.46 | 69.09,29.46 v66.42,29.46 | v46.23,44.85 v46.23,36.07 46.16,36.13 40.2,36.13 39.75,36.58 38.54,36.58 v38.16,36.2 | v58.17,44.83 v58.17,37.59 56.52,37.59 54.99,36.07 v54.99,35.56 v54.99,29.34 v58.67,29.34
  Bottom 0.406: C14.+ 16.19,25.39 v16.19,34.67

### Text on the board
tNames: EBC | amp_neg | gnd | pll_dc | pll_attn | amp_neg | gnd | pll_in | -18V | pot_tap | pot_tap | pot_1 | pot_tap | -18v | 0V | pot_1 | pot_vss | gnd | +5V | +18V | 2nd | 1st | BYU Holography / 10 Mar 2015 | Dr. Daniel Smalley / Andrew Henrie
Document: 6 June 2015: / The only mistake discovered on this board / to date is that this wire wasn't routed. / This has now been fixed in the .brd and / gerber files, but double-check your board. / If it is missing, make this connection; the / board works after doing this. / - Andrew Henrie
